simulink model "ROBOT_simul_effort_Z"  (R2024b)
settings: Solver=VariableStepAuto  StartTime=0.0  StopTime=5  RelTol=1e-3
undefined symbols (not defined in the file): a, ARRIERE_Defaut_sldprt, avant01_Defaut_sldprt, avant02_Defaut_sldprt, avant03_Defaut_sldprt, avant1_Defaut_sldprt, AXE, BASE_Defaut_sldprt, BIELLE, BIELLE_Defaut_sldprt, BRAS_Defaut_sldprt, bras_Defaut_sldprt, C_Realiste_sldprt, CABLE_Defaut_sldprt, cable_Defaut_sldprt, CACHE_Defaut_sldprt, CARTE, carte_Defaut_sldprt, CARTER, carter, CHC, CODEUR_Defaut_sldprt, cruciforme, cylindrique, deg, Drive, Fichiers, Fichiers_Matlab_sujetA, FIXATION, fixation_Defaut_sldprt, H, HEXAGONALE_Defaut_sldprt, joint_Defaut_sldprt, kg, m, M4, M4_Defaut_sldprt, manette1_Defaut_sldprt, manette2_Defaut_sldprt, MATLAB, Matlab, matlab_Defaut_sldprt, mm, modif, MOTEUR_Defaut_sldprt, N, NEZ_Defaut_sldprt, nom, palier, PARALLELOGRAMME_Defaut_sldprt, petite, plaque, rad, Ressort, Rondelle, ROTOR_Defaut_sldprt, s, SET, simple, socle_Defaut_sldprt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
libraries: sm_lib x463, fl_lib x45, nesl_utility x27, simulink x2
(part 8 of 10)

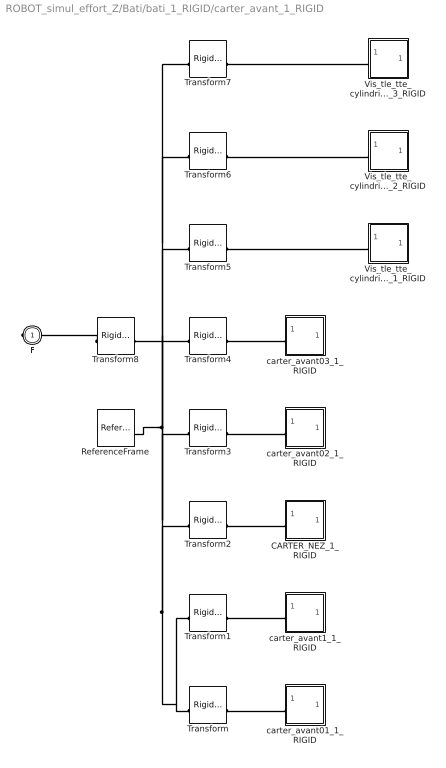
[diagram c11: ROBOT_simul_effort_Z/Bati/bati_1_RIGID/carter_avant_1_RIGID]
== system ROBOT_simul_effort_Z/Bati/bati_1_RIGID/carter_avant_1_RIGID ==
  CARTER_NEZ_1_RIGID : Subsystem
  ReferenceFrame : sm_lib/Frames and Transforms/Reference Frame
  Transform : sm_lib/Frames and Transforms/Rigid Transform  RotationMethod=None  FollAlignAxisA=+X  BaseAlignAxisA=+Y  FollAlignAxisB=+Y  BaseAlignAxisB=+Z  RotationStandardAxis=+Z  RotationAngle=0  RotationAngleUnits=deg  RotationArbitraryAxis=[0 0 1]  RotationSequenceAxes=FollowerAxes  RotationSequence=XYX  RotationSequenceAngles=[0 0 0]  RotationSequenceAnglesUnits=deg  RotationMatrix=[1 0 0; 0 1 0; 0 0 1]  Quaternion=[1 0 0 0]  TranslationMethod=Cartesian  TranslationCartesianOffset=[-17.102622676542445 -113.90982355031112 -1.7985612998927536e-11]  TranslationCartesianOffsetUnits=mm  TranslationStandardAxis=+Z  TranslationStandardOffset=0  TranslationStandardOffsetUnits=mm  TranslationROffset=0  TranslationROffsetUnits=m  TranslationThetaOffset=0  TranslationThetaOffsetUnits=deg  TranslationZOffset=0  TranslationZOffsetUnits=m
  Transform1 : sm_lib/Frames and Transforms/Rigid Transform  RotationMethod=None  FollAlignAxisA=+X  BaseAlignAxisA=+Y  FollAlignAxisB=+Y  BaseAlignAxisB=+Z  RotationStandardAxis=+Z  RotationAngle=0  RotationAngleUnits=deg  RotationArbitraryAxis=[0 0 1]  RotationSequenceAxes=FollowerAxes  RotationSequence=XYX  RotationSequenceAngles=[0 0 0]  RotationSequenceAnglesUnits=deg  RotationMatrix=[1 0 0; 0 1 0; 0 0 1]  Quaternion=[1 0 0 0]  TranslationMethod=Cartesian  TranslationCartesianOffset=[-17.102622676541863 -113.90982355031173 -1.7985612998927536e-11]  TranslationCartesianOffsetUnits=mm  TranslationStandardAxis=+Z  TranslationStandardOffset=0  TranslationStandardOffsetUnits=mm  TranslationROffset=0  TranslationROffsetUnits=m  TranslationThetaOffset=0  TranslationThetaOffsetUnits=deg  TranslationZOffset=0  TranslationZOffsetUnits=m
  Transform2 : sm_lib/Frames and Transforms/Rigid Transform  RotationMethod=ArbitraryAxis  FollAlignAxisA=+X  BaseAlignAxisA=+Y  FollAlignAxisB=+Y  BaseAlignAxisB=+Z  RotationStandardAxis=+Z  RotationAngle=3.1415926535897931  RotationAngleUnits=rad  RotationArbitraryAxis=[0 0.70710678118654746 0.70710678118654757]  RotationSequenceAxes=FollowerAxes  RotationSequence=XYX  RotationSequenceAngles=[0 0 0]  RotationSequenceAnglesUnits=deg  RotationMatrix=[1 0 0; 0 1 0; 0 0 1]  Quaternion=[1 0 0 0]  TranslationMethod=None  TranslationCartesianOffset=[0 0 0]  TranslationCartesianOffsetUnits=m  TranslationStandardAxis=+Z  TranslationStandardOffset=0  TranslationStandardOffsetUnits=m  TranslationROffset=0  TranslationROffsetUnits=m  TranslationThetaOffset=0  TranslationThetaOffsetUnits=deg  TranslationZOffset=0  TranslationZOffsetUnits=m
  Transform3 : sm_lib/Frames and Transforms/Rigid Transform  RotationMethod=ArbitraryAxis  FollAlignAxisA=+X  BaseAlignAxisA=+Y  FollAlignAxisB=+Y  BaseAlignAxisB=+Z  RotationStandardAxis=+Z  RotationAngle=2.094395102393193  RotationAngleUnits=rad  RotationArbitraryAxis=[0 0 1]  RotationSequenceAxes=FollowerAxes  RotationSequence=XYX  RotationSequenceAngles=[0 0 0]  RotationSequenceAnglesUnits=deg  RotationMatrix=[1 0 0; 0 1 0; 0 0 1]  Quaternion=[1 0 0 0]  TranslationMethod=Cartesian  TranslationCartesianOffset=[82.706805109614251 58.965176449688634 -1.7985612998927536e-11]  TranslationCartesianOffsetUnits=mm  TranslationStandardAxis=+Z  TranslationStandardOffset=0  TranslationStandardOffsetUnits=mm  TranslationROffset=0  TranslationROffsetUnits=m  TranslationThetaOffset=0  TranslationThetaOffsetUnits=deg  TranslationZOffset=0  TranslationZOffsetUnits=m
  Transform4 : sm_lib/Frames and Transforms/Rigid Transform  RotationMethod=ArbitraryAxis  FollAlignAxisA=+X  BaseAlignAxisA=+Y  FollAlignAxisB=+Y  BaseAlignAxisB=+Z  RotationStandardAxis=+Z  RotationAngle=2.0943951023932006  RotationAngleUnits=rad  RotationArbitraryAxis=[-0 -0 -1]  RotationSequenceAxes=FollowerAxes  RotationSequence=XYX  RotationSequenceAngles=[0 0 0]  RotationSequenceAnglesUnits=deg  RotationMatrix=[1 0 0; 0 1 0; 0 0 1]  Quaternion=[1 0 0 0]  TranslationMethod=Cartesian  TranslationCartesianOffset=[-116.91205046269873 58.965176449689402 -1.7985612998927536e-11]  TranslationCartesianOffsetUnits=mm  TranslationStandardAxis=+Z  TranslationStandardOffset=0  TranslationStandardOffsetUnits=mm  TranslationROffset=0  TranslationROffsetUnits=m  TranslationThetaOffset=0  TranslationThetaOffsetUnits=deg  TranslationZOffset=0  TranslationZOffsetUnits=m
  Transform5 : sm_lib/Frames and Transforms/Rigid Transform  RotationMethod=ArbitraryAxis  FollAlignAxisA=+X  BaseAlignAxisA=+Y  FollAlignAxisB=+Y  BaseAlignAxisB=+Z  RotationStandardAxis=+Z  RotationAngle=1.5707963267948968  RotationAngleUnits=rad  RotationArbitraryAxis=[0 1 0]  RotationSequenceAxes=FollowerAxes  RotationSequence=XYX  RotationSequenceAngles=[0 0 0]  RotationSequenceAnglesUnits=deg  RotationMatrix=[1 0 0; 0 1 0; 0 0 1]  Quaternion=[1 0 0 0]  TranslationMethod=Cartesian  TranslationCartesianOffset=[-32.01022121330513 -41.991412127562512 96.999999999981995]  TranslationCartesianOffsetUnits=mm  TranslationStandardAxis=+Z  TranslationStandardOffset=0  TranslationStandardOffsetUnits=mm  TranslationROffset=0  TranslationROffsetUnits=m  TranslationThetaOffset=0  TranslationThetaOffsetUnits=deg  TranslationZOffset=0  TranslationZOffsetUnits=m
  Transform6 : sm_lib/Frames and Transforms/Rigid Transform  RotationMethod=ArbitraryAxis  FollAlignAxisA=+X  BaseAlignAxisA=+Y  FollAlignAxisB=+Y  BaseAlignAxisB=+Z  RotationStandardAxis=+Z  RotationAngle=1.5707963267948968  RotationAngleUnits=rad  RotationArbitraryAxis=[0 1 0]  RotationSequenceAxes=FollowerAxes  RotationSequence=XYX  RotationSequenceAngles=[0 0 0]  RotationSequenceAnglesUnits=deg  RotationMatrix=[1 0 0; 0 1 0; 0 0 1]  Quaternion=[1 0 0 0]  TranslationMethod=Cartesian  TranslationCartesianOffset=[-47.17507990239649 35.916329780570692 96.999999999981995]  TranslationCartesianOffsetUnits=mm  TranslationStandardAxis=+Z  TranslationStandardOffset=0  TranslationStandardOffsetUnits=mm  TranslationROffset=0  TranslationROffsetUnits=m  TranslationThetaOffset=0  TranslationThetaOffsetUnits=deg  TranslationZOffset=0  TranslationZOffsetUnits=m
  Transform7 : sm_lib/Frames and Transforms/Rigid Transform  RotationMethod=ArbitraryAxis  FollAlignAxisA=+X  BaseAlignAxisA=+Y  FollAlignAxisB=+Y  BaseAlignAxisB=+Z  RotationStandardAxis=+Z  RotationAngle=1.5707963267948968  RotationAngleUnits=rad  RotationArbitraryAxis=[0 1 0]  RotationSequenceAxes=FollowerAxes  RotationSequence=XYX  RotationSequenceAngles=[0 0 0]  RotationSequenceAnglesUnits=deg  RotationMatrix=[1 0 0; 0 1 0; 0 0 1]  Quaternion=[1 0 0 0]  TranslationMethod=Cartesian  TranslationCartesianOffset=[27.877433086074202 10.09561169605827 96.999999999981995]  TranslationCartesianOffsetUnits=mm  TranslationStandardAxis=+Z  TranslationStandardOffset=0  TranslationStandardOffsetUnits=mm  TranslationROffset=0  TranslationROffsetUnits=m  TranslationThetaOffset=0  TranslationThetaOffsetUnits=deg  TranslationZOffset=0  TranslationZOffsetUnits=m
  Transform8 : sm_lib/Frames and Transforms/Rigid Transform  RotationMethod=None  FollAlignAxisA=+X  BaseAlignAxisA=+Y  FollAlignAxisB=+Y  BaseAlignAxisB=+Z  RotationStandardAxis=+Z  RotationAngle=0  RotationAngleUnits=deg  RotationArbitraryAxis=[0 0 1]  RotationSequenceAxes=FollowerAxes  RotationSequence=XYX  RotationSequenceAngles=[0 0 0]  RotationSequenceAnglesUnits=deg  RotationMatrix=[1 0 0; 0 1 0; 0 0 1]  Quaternion=[1 0 0 0]  TranslationMethod=Cartesian  TranslationCartesianOffset=[17.102622676542548 113.90982355031109 24.00000000001798]  TranslationCartesianOffsetUnits=mm  TranslationStandardAxis=+Z  TranslationStandardOffset=0  TranslationStandardOffsetUnits=mm  TranslationROffset=0  TranslationROffsetUnits=m  TranslationThetaOffset=0  TranslationThetaOffsetUnits=deg  TranslationZOffset=0  TranslationZOffsetUnits=m
  Vis_tle_tte_cylindrique_cruciforme_H_29x13_C_1_RIGID : Subsystem
  Vis_tle_tte_cylindrique_cruciforme_H_29x13_C_2_RIGID : Subsystem
  Vis_tle_tte_cylindrique_cruciforme_H_29x13_C_3_RIGID : Subsystem
  carter_avant01_1_RIGID : Subsystem
  carter_avant02_1_RIGID : Subsystem
  carter_avant03_1_RIGID : Subsystem
  carter_avant1_1_RIGID : Subsystem
  F : PMIOPort  Side=Right
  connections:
  Transform/RConn1 -- carter_avant01_1_RIGID/LConn1
  Transform1/RConn1 -- carter_avant1_1_RIGID/LConn1
  CARTER_NEZ_1_RIGID/LConn1 -- Transform2/RConn1
  Transform3/RConn1 -- carter_avant02_1_RIGID/LConn1
  Transform4/RConn1 -- carter_avant03_1_RIGID/LConn1
  Transform5/RConn1 -- Vis_tle_tte_cylindrique_cruciforme_H_29x13_C_1_RIGID/LConn1
  Transform6/RConn1 -- Vis_tle_tte_cylindrique_cruciforme_H_29x13_C_2_RIGID/LConn1
  Transform7/RConn1 -- Vis_tle_tte_cylindrique_cruciforme_H_29x13_C_3_RIGID/LConn1
  Transform/LConn1 -- Transform6/LConn1 -- Transform7/LConn1 -- Transform5/LConn1 -- Transform4/LConn1 -- ReferenceFrame/RConn1 -- Transform8/RConn1 -- Transform3/LConn1 -- Transform2/LConn1 -- Transform1/LConn1
  Transform8/LConn1 -- F/RConn1

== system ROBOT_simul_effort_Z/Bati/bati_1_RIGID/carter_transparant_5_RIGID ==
  ReferenceFrame : sm_lib/Frames and Transforms/Reference Frame
  Transform : sm_lib/Frames and Transforms/Rigid Transform  RotationMethod=ArbitraryAxis  FollAlignAxisA=+X  BaseAlignAxisA=+Y  FollAlignAxisB=+Y  BaseAlignAxisB=+Z  RotationStandardAxis=+Z  RotationAngle=2.0943951023932001  RotationAngleUnits=rad  RotationArbitraryAxis=[-0 -0 -1]  RotationSequenceAxes=FollowerAxes  RotationSequence=XYX  RotationSequenceAngles=[0 0 0]  RotationSequenceAnglesUnits=deg  RotationMatrix=[1 0 0; 0 1 0; 0 0 1]  Quaternion=[1 0 0 0]  TranslationMethod=Cartesian  TranslationCartesianOffset=[-114.07592590479371 112.90132228455712 35.212494571905935]  TranslationCartesianOffsetUnits=mm  TranslationStandardAxis=+Z  TranslationStandardOffset=0  TranslationStandardOffsetUnits=mm  TranslationROffset=0  TranslationROffsetUnits=m  TranslationThetaOffset=0  TranslationThetaOffsetUnits=deg  TranslationZOffset=0  TranslationZOffsetUnits=m
  Transform1 : sm_lib/Frames and Transforms/Rigid Transform  RotationMethod=None  FollAlignAxisA=+X  BaseAlignAxisA=+Y  FollAlignAxisB=+Y  BaseAlignAxisB=+Z  RotationStandardAxis=+Z  RotationAngle=0  RotationAngleUnits=deg  RotationArbitraryAxis=[0 0 1]  RotationSequenceAxes=FollowerAxes  RotationSequence=XYX  RotationSequenceAngles=[0 0 0]  RotationSequenceAnglesUnits=deg  RotationMatrix=[1 0 0; 0 1 0; 0 0 1]  Quaternion=[1 0 0 0]  TranslationMethod=Cartesian  TranslationCartesianOffset=[-14.266498118637394 -59.973677715443351 35.212494571905921]  TranslationCartesianOffsetUnits=mm  TranslationStandardAxis=+Z  TranslationStandardOffset=0  TranslationStandardOffsetUnits=mm  TranslationROffset=0  TranslationROffsetUnits=m  TranslationThetaOffset=0  TranslationThetaOffsetUnits=deg  TranslationZOffset=0  TranslationZOffsetUnits=m
  Transform2 : sm_lib/Frames and Transforms/Rigid Transform  RotationMethod=ArbitraryAxis  FollAlignAxisA=+X  BaseAlignAxisA=+Y  FollAlignAxisB=+Y  BaseAlignAxisB=+Z  RotationStandardAxis=+Z  RotationAngle=2.0943951023931877  RotationAngleUnits=rad  RotationArbitraryAxis=[0 0 1]  RotationSequenceAxes=FollowerAxes  RotationSequence=XYX  RotationSequenceAngles=[0 0 0]  RotationSequenceAnglesUnits=deg  RotationMatrix=[1 0 0; 0 1 0; 0 0 1]  Quaternion=[1 0 0 0]  TranslationMethod=Cartesian  TranslationCartesianOffset=[85.542929667519687 112.90132228455593 35.212494571905921]  TranslationCartesianOffsetUnits=mm  TranslationStandardAxis=+Z  TranslationStandardOffset=0  TranslationStandardOffsetUnits=mm  TranslationROffset=0  TranslationROffsetUnits=m  TranslationThetaOffset=0  TranslationThetaOffsetUnits=deg  TranslationZOffset=0  TranslationZOffsetUnits=m
  Transform3 : sm_lib/Frames and Transforms/Rigid Transform  RotationMethod=ArbitraryAxis  FollAlignAxisA=+X  BaseAlignAxisA=+Y  FollAlignAxisB=+Y  BaseAlignAxisB=+Z  RotationStandardAxis=+Z  RotationAngle=0.025132741228718395  RotationAngleUnits=rad  RotationArbitraryAxis=[0 0 -1]  RotationSequenceAxes=FollowerAxes  RotationSequence=XYX  RotationSequenceAngles=[0 0 0]  RotationSequenceAnglesUnits=deg  RotationMatrix=[1 0 0; 0 1 0; 0 0 1]  Quaternion=[1 0 0 0]  TranslationMethod=Cartesian  TranslationCartesianOffset=[12.872893350874152 59.632616111037024 -35.212494571905921]  TranslationCartesianOffsetUnits=mm  TranslationStandardAxis=+Z  TranslationStandardOffset=0  TranslationStandardOffsetUnits=mm  TranslationROffset=0  TranslationROffsetUnits=m  TranslationThetaOffset=0  TranslationThetaOffsetUnits=deg  TranslationZOffset=0  TranslationZOffsetUnits=m
  carter_transparent2_1_RIGID : Subsystem
  carter_transparent_1_RIGID : Subsystem
  carter_transparent_modif_matlab_1_RIGID : Subsystem
  F : PMIOPort  Side=Right
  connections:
  Transform/RConn1 -- carter_transparent_1_RIGID/LConn1
  Transform1/RConn1 -- carter_transparent2_1_RIGID/LConn1
  Transform2/RConn1 -- carter_transparent_modif_matlab_1_RIGID/LConn1
  Transform/LConn1 -- Transform1/LConn1 -- Transform2/LConn1 -- ReferenceFrame/RConn1 -- Transform3/RConn1
  Transform3/LConn1 -- F/RConn1

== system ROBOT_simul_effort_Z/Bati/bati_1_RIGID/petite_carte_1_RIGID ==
  ReferenceFrame : sm_lib/Frames and Transforms/Reference Frame
  Solid : sm_lib/Body Elements/File Solid  ExtGeomFileName=/MATLAB Drive/Fichiers_Matlab_sujetA/Fichiers Matlab/STL/petite carte_Defaut_sldprt.STL  UnitType=Custom  ExtGeomFileUnits=mm  StepReaderType=HEX  ExportConvexHullGeometry=off  InertiaType=Custom  BasedOnType=Density  Density=1000  DensityUnits=kg/(m^3)  Mass=0.00048082183649251445  MassUnits=kg  CenterOfMass=[19.91458998704724 1.4286045215267169 0.6668228749994265]  CenterOfMassUnits=mm  MomentsOfInertia=[0.0075326471062909569 0.048633515547401453 0.053492974016950315]  MomentsOfInertiaUnits=kg*mm^2  ProductsOfInertia=[9.9546833043094831e-05 0.0011485008863759011 0.0086575785704640102]  ProductsOfInertiaUnits=kg*mm^2  GraphicType=FromGeometry  MarkerShape=Sphere  MarkerSize=10  GraphicVisPropType=SimpleVisualProperties  GraphicDiffuseColor=[0 0.50196078431372548 0]  GraphicOpacity=1  GraphicSpecularColor=[0.5 0.5 0.5 1.0]  GraphicAmbientColor=[0.15 0.15 0.15 1.0]  GraphicEmissiveColor=[0.0 0.0 0.0 1.0]  GraphicShininess=75  DoExposeReferenceFrame=on  SerializedFrames=<Frames/>
  F : PMIOPort  Side=Left
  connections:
  Solid/RConn1 -- ReferenceFrame/RConn1 -- F/RConn1

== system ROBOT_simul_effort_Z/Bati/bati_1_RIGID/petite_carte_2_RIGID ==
  ReferenceFrame : sm_lib/Frames and Transforms/Reference Frame
  Solid : sm_lib/Body Elements/File Solid  ExtGeomFileName=/MATLAB Drive/Fichiers_Matlab_sujetA/Fichiers Matlab/STL/petite carte_Defaut_sldprt.STL  UnitType=Custom  ExtGeomFileUnits=mm  StepReaderType=HEX  ExportConvexHullGeometry=off  InertiaType=Custom  BasedOnType=Density  Density=1000  DensityUnits=kg/(m^3)  Mass=0.00048082183649251445  MassUnits=kg  CenterOfMass=[19.91458998704724 1.4286045215267169 0.6668228749994265]  CenterOfMassUnits=mm  MomentsOfInertia=[0.0075326471062909569 0.048633515547401453 0.053492974016950315]  MomentsOfInertiaUnits=kg*mm^2  ProductsOfInertia=[9.9546833043094831e-05 0.0011485008863759011 0.0086575785704640102]  ProductsOfInertiaUnits=kg*mm^2  GraphicType=FromGeometry  MarkerShape=Sphere  MarkerSize=10  GraphicVisPropType=SimpleVisualProperties  GraphicDiffuseColor=[0 0.50196078431372548 0]  GraphicOpacity=1  GraphicSpecularColor=[0.5 0.5 0.5 1.0]  GraphicAmbientColor=[0.15 0.15 0.15 1.0]  GraphicEmissiveColor=[0.0 0.0 0.0 1.0]  GraphicShininess=75  DoExposeReferenceFrame=on  SerializedFrames=<Frames/>
  F : PMIOPort  Side=Left
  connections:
  Solid/RConn1 -- ReferenceFrame/RConn1 -- F/RConn1

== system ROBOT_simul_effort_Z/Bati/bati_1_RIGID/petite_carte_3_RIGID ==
  ReferenceFrame : sm_lib/Frames and Transforms/Reference Frame
  Solid : sm_lib/Body Elements/File Solid  ExtGeomFileName=/MATLAB Drive/Fichiers_Matlab_sujetA/Fichiers Matlab/STL/petite carte_Defaut_sldprt.STL  UnitType=Custom  ExtGeomFileUnits=mm  StepReaderType=HEX  ExportConvexHullGeometry=off  InertiaType=Custom  BasedOnType=Density  Density=1000  DensityUnits=kg/(m^3)  Mass=0.00048082183649251445  MassUnits=kg  CenterOfMass=[19.91458998704724 1.4286045215267169 0.6668228749994265]  CenterOfMassUnits=mm  MomentsOfInertia=[0.0075326471062909569 0.048633515547401453 0.053492974016950315]  MomentsOfInertiaUnits=kg*mm^2  ProductsOfInertia=[9.9546833043094831e-05 0.0011485008863759011 0.0086575785704640102]  ProductsOfInertiaUnits=kg*mm^2  GraphicType=FromGeometry  MarkerShape=Sphere  MarkerSize=10  GraphicVisPropType=SimpleVisualProperties  GraphicDiffuseColor=[0 0.50196078431372548 0]  GraphicOpacity=1  GraphicSpecularColor=[0.5 0.5 0.5 1.0]  GraphicAmbientColor=[0.15 0.15 0.15 1.0]  GraphicEmissiveColor=[0.0 0.0 0.0 1.0]  GraphicShininess=75  DoExposeReferenceFrame=on  SerializedFrames=<Frames/>
  F : PMIOPort  Side=Left
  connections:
  Solid/RConn1 -- ReferenceFrame/RConn1 -- F/RConn1

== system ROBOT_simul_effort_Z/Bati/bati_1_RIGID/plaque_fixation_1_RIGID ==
  ReferenceFrame : sm_lib/Frames and Transforms/Reference Frame
  Solid : sm_lib/Body Elements/File Solid  ExtGeomFileName=/MATLAB Drive/Fichiers_Matlab_sujetA/Fichiers Matlab/STL/plaque fixation_Defaut_sldprt.STL  UnitType=Custom  ExtGeomFileUnits=mm  StepReaderType=HEX  ExportConvexHullGeometry=off  InertiaType=Custom  BasedOnType=Density  Density=1000  DensityUnits=kg/(m^3)  Mass=0.13619587212093154  MassUnits=kg  CenterOfMass=[0 57.644814512190067 6.7752904956014124]  CenterOfMassUnits=mm  MomentsOfInertia=[230.56748251711528 59.503021506275417 273.91192419339654]  MomentsOfInertiaUnits=kg*mm^2  ProductsOfInertia=[16.91481201365259 0 0]  ProductsOfInertiaUnits=kg*mm^2  GraphicType=FromGeometry  MarkerShape=Sphere  MarkerSize=10  GraphicVisPropType=SimpleVisualProperties  GraphicDiffuseColor=[0.6470588235294118 0.61960784313725492 0.58823529411764708]  GraphicOpacity=1  GraphicSpecularColor=[0.5 0.5 0.5 1.0]  GraphicAmbientColor=[0.15 0.15 0.15 1.0]  GraphicEmissiveColor=[0.0 0.0 0.0 1.0]  GraphicShininess=75  DoExposeReferenceFrame=on  SerializedFrames=<Frames/>
  F : PMIOPort  Side=Left
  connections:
  Solid/RConn1 -- ReferenceFrame/RConn1 -- F/RConn1

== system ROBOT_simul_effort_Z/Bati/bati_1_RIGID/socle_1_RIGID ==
  ReferenceFrame : sm_lib/Frames and Transforms/Reference Frame
  Solid : sm_lib/Body Elements/File Solid  ExtGeomFileName=/MATLAB Drive/Fichiers_Matlab_sujetA/Fichiers Matlab/STL/socle_Defaut_sldprt.STL  UnitType=Custom  ExtGeomFileUnits=mm  StepReaderType=HEX  ExportConvexHullGeometry=off  InertiaType=Custom  BasedOnType=Density  Density=1000  DensityUnits=kg/(m^3)  Mass=0.22494978957848721  MassUnits=kg  CenterOfMass=[-0.04792533570938888 16.018647482078187 6.7264124950212594]  CenterOfMassUnits=mm  MomentsOfInertia=[992.11143480501664 1618.7630611955949 2601.3810500563377]  MomentsOfInertiaUnits=kg*mm^2  ProductsOfInertia=[-5.1990662975402211 -0.041150083489637494 0.38689094335060764]  ProductsOfInertiaUnits=kg*mm^2  GraphicType=FromGeometry  MarkerShape=Sphere  MarkerSize=10  GraphicVisPropType=SimpleVisualProperties  GraphicDiffuseColor=[0.792156862745098 0.81960784313725488 0.93333333333333335]  GraphicOpacity=1  GraphicSpecularColor=[0.5 0.5 0.5 1.0]  GraphicAmbientColor=[0.15 0.15 0.15 1.0]  GraphicEmissiveColor=[0.0 0.0 0.0 1.0]  GraphicShininess=75  DoExposeReferenceFrame=on  SerializedFrames=<Frames/>
  F : PMIOPort  Side=Left
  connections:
  Solid/RConn1 -- ReferenceFrame/RConn1 -- F/RConn1

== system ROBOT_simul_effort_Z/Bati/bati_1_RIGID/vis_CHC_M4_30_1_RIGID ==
  ReferenceFrame : sm_lib/Frames and Transforms/Reference Frame
  Solid : sm_lib/Body Elements/File Solid  ExtGeomFileName=/MATLAB Drive/Fichiers_Matlab_sujetA/Fichiers Matlab/STL/vis CHC M4-30_Defaut_sldprt.STL  UnitType=Custom  ExtGeomFileUnits=mm  StepReaderType=HEX  ExportConvexHullGeometry=off  InertiaType=Custom  BasedOnType=Density  Density=1000  DensityUnits=kg/(m^3)  Mass=0.00050829612748328964  MassUnits=kg  CenterOfMass=[0 0 19.413574172112984]  CenterOfMassUnits=mm  MomentsOfInertia=[0.056747582392929367 0.056747582392929367 0.0016443905083794684]  MomentsOfInertiaUnits=kg*mm^2  ProductsOfInertia=[0 0 0]  ProductsOfInertiaUnits=kg*mm^2  GraphicType=FromGeometry  MarkerShape=Sphere  MarkerSize=10  GraphicVisPropType=SimpleVisualProperties  GraphicDiffuseColor=[0.75294117647058822 0.75294117647058822 0.75294117647058822]  GraphicOpacity=1  GraphicSpecularColor=[0.5 0.5 0.5 1.0]  GraphicAmbientColor=[0.15 0.15 0.15 1.0]  GraphicEmissiveColor=[0.0 0.0 0.0 1.0]  GraphicShininess=75  DoExposeReferenceFrame=on  SerializedFrames=<Frames/>
  F : PMIOPort  Side=Left
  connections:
  Solid/RConn1 -- ReferenceFrame/RConn1 -- F/RConn1

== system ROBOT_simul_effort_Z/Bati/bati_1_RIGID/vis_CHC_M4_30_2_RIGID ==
  ReferenceFrame : sm_lib/Frames and Transforms/Reference Frame
  Solid : sm_lib/Body Elements/File Solid  ExtGeomFileName=/MATLAB Drive/Fichiers_Matlab_sujetA/Fichiers Matlab/STL/vis CHC M4-30_Defaut_sldprt.STL  UnitType=Custom  ExtGeomFileUnits=mm  StepReaderType=HEX  ExportConvexHullGeometry=off  InertiaType=Custom  BasedOnType=Density  Density=1000  DensityUnits=kg/(m^3)  Mass=0.00050829612748328964  MassUnits=kg  CenterOfMass=[0 0 19.413574172112984]  CenterOfMassUnits=mm  MomentsOfInertia=[0.056747582392929367 0.056747582392929367 0.0016443905083794684]  MomentsOfInertiaUnits=kg*mm^2  ProductsOfInertia=[0 0 0]  ProductsOfInertiaUnits=kg*mm^2  GraphicType=FromGeometry  MarkerShape=Sphere  MarkerSize=10  GraphicVisPropType=SimpleVisualProperties  GraphicDiffuseColor=[0.75294117647058822 0.75294117647058822 0.75294117647058822]  GraphicOpacity=1  GraphicSpecularColor=[0.5 0.5 0.5 1.0]  GraphicAmbientColor=[0.15 0.15 0.15 1.0]  GraphicEmissiveColor=[0.0 0.0 0.0 1.0]  GraphicShininess=75  DoExposeReferenceFrame=on  SerializedFrames=<Frames/>
  F : PMIOPort  Side=Left
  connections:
  Solid/RConn1 -- ReferenceFrame/RConn1 -- F/RConn1

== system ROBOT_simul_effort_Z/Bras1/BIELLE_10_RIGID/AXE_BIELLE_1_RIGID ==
  ReferenceFrame : sm_lib/Frames and Transforms/Reference Frame
  Solid : sm_lib/Body Elements/File Solid  ExtGeomFileName=/MATLAB Drive/Fichiers_Matlab_sujetA/Fichiers Matlab/STL/AXE BIELLE_Defaut_sldprt.STL  UnitType=Custom  ExtGeomFileUnits=mm  StepReaderType=HEX  ExportConvexHullGeometry=off  InertiaType=Custom  BasedOnType=Density  Density=1000  DensityUnits=kg/(m^3)  Mass=0.0008880235381781051  MassUnits=kg  CenterOfMass=[0 0 0]  CenterOfMassUnits=mm  MomentsOfInertia=[0.018768660222737772 0.018768660222737772 0.0009874025874388381]  MomentsOfInertiaUnits=kg*mm^2  ProductsOfInertia=[0 0 0]  ProductsOfInertiaUnits=kg*mm^2  GraphicType=FromGeometry  MarkerShape=Sphere  MarkerSize=10  GraphicVisPropType=SimpleVisualProperties  GraphicDiffuseColor=[1 0.94901960784313721 0.90980392156862744]  GraphicOpacity=1  GraphicSpecularColor=[0.5 0.5 0.5 1.0]  GraphicAmbientColor=[0.15 0.15 0.15 1.0]  GraphicEmissiveColor=[0.0 0.0 0.0 1.0]  GraphicShininess=75  DoExposeReferenceFrame=on  SerializedFrames=<Frames/>
  F : PMIOPort  Side=Left
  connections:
  Solid/RConn1 -- ReferenceFrame/RConn1 -- F/RConn1

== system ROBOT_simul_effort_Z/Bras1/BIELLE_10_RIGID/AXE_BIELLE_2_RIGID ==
  ReferenceFrame : sm_lib/Frames and Transforms/Reference Frame
  Solid : sm_lib/Body Elements/File Solid  ExtGeomFileName=/MATLAB Drive/Fichiers_Matlab_sujetA/Fichiers Matlab/STL/AXE BIELLE_Defaut_sldprt.STL  UnitType=Custom  ExtGeomFileUnits=mm  StepReaderType=HEX  ExportConvexHullGeometry=off  InertiaType=Custom  BasedOnType=Density  Density=1000  DensityUnits=kg/(m^3)  Mass=0.0008880235381781051  MassUnits=kg  CenterOfMass=[0 0 0]  CenterOfMassUnits=mm  MomentsOfInertia=[0.018768660222737772 0.018768660222737772 0.0009874025874388381]  MomentsOfInertiaUnits=kg*mm^2  ProductsOfInertia=[0 0 0]  ProductsOfInertiaUnits=kg*mm^2  GraphicType=FromGeometry  MarkerShape=Sphere  MarkerSize=10  GraphicVisPropType=SimpleVisualProperties  GraphicDiffuseColor=[1 0.94901960784313721 0.90980392156862744]  GraphicOpacity=1  GraphicSpecularColor=[0.5 0.5 0.5 1.0]  GraphicAmbientColor=[0.15 0.15 0.15 1.0]  GraphicEmissiveColor=[0.0 0.0 0.0 1.0]  GraphicShininess=75  DoExposeReferenceFrame=on  SerializedFrames=<Frames/>
  F : PMIOPort  Side=Left
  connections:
  Solid/RConn1 -- ReferenceFrame/RConn1 -- F/RConn1

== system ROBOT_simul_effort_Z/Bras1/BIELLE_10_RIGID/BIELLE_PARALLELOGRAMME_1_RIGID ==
  ReferenceFrame : sm_lib/Frames and Transforms/Reference Frame
  Solid : sm_lib/Body Elements/File Solid  ExtGeomFileName=/MATLAB Drive/Fichiers_Matlab_sujetA/Fichiers Matlab/STL/BIELLE PARALLELOGRAMME_Defaut_sldprt.STL  UnitType=Custom  ExtGeomFileUnits=mm  StepReaderType=HEX  ExportConvexHullGeometry=off  InertiaType=Custom  BasedOnType=Density  Density=1000  DensityUnits=kg/(m^3)  Mass=0.0079529027635324764  MassUnits=kg  CenterOfMass=[0 3.1653377955585489 0]  CenterOfMassUnits=mm  MomentsOfInertia=[7.7987017961340088 7.8475939194203406 0.14816857834406802]  MomentsOfInertiaUnits=kg*mm^2  ProductsOfInertia=[0 0 0]  ProductsOfInertiaUnits=kg*mm^2  GraphicType=FromGeometry  MarkerShape=Sphere  MarkerSize=10  GraphicVisPropType=SimpleVisualProperties  GraphicDiffuseColor=[0.6 1.0 1.0]  GraphicOpacity=1  GraphicSpecularColor=[0.5 0.5 0.5 1.0]  GraphicAmbientColor=[0.15 0.15 0.15 1.0]  GraphicEmissiveColor=[0.0 0.0 0.0 1.0]  GraphicShininess=75  DoExposeReferenceFrame=on  SerializedFrames=<Frames/>
  F : PMIOPort  Side=Left
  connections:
  Solid/RConn1 -- ReferenceFrame/RConn1 -- F/RConn1

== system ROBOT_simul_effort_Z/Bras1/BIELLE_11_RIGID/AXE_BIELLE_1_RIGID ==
  ReferenceFrame : sm_lib/Frames and Transforms/Reference Frame
  Solid : sm_lib/Body Elements/File Solid  ExtGeomFileName=/MATLAB Drive/Fichiers_Matlab_sujetA/Fichiers Matlab/STL/AXE BIELLE_Defaut_sldprt.STL  UnitType=Custom  ExtGeomFileUnits=mm  StepReaderType=HEX  ExportConvexHullGeometry=off  InertiaType=Custom  BasedOnType=Density  Density=1000  DensityUnits=kg/(m^3)  Mass=0.0008880235381781051  MassUnits=kg  CenterOfMass=[0 0 0]  CenterOfMassUnits=mm  MomentsOfInertia=[0.018768660222737772 0.018768660222737772 0.0009874025874388381]  MomentsOfInertiaUnits=kg*mm^2  ProductsOfInertia=[0 0 0]  ProductsOfInertiaUnits=kg*mm^2  GraphicType=FromGeometry  MarkerShape=Sphere  MarkerSize=10  GraphicVisPropType=SimpleVisualProperties  GraphicDiffuseColor=[1 0.94901960784313721 0.90980392156862744]  GraphicOpacity=1  GraphicSpecularColor=[0.5 0.5 0.5 1.0]  GraphicAmbientColor=[0.15 0.15 0.15 1.0]  GraphicEmissiveColor=[0.0 0.0 0.0 1.0]  GraphicShininess=75  DoExposeReferenceFrame=on  SerializedFrames=<Frames/>
  F : PMIOPort  Side=Left
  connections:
  Solid/RConn1 -- ReferenceFrame/RConn1 -- F/RConn1

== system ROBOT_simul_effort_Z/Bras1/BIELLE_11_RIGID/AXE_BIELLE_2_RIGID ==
  ReferenceFrame : sm_lib/Frames and Transforms/Reference Frame
  Solid : sm_lib/Body Elements/File Solid  ExtGeomFileName=/MATLAB Drive/Fichiers_Matlab_sujetA/Fichiers Matlab/STL/AXE BIELLE_Defaut_sldprt.STL  UnitType=Custom  ExtGeomFileUnits=mm  StepReaderType=HEX  ExportConvexHullGeometry=off  InertiaType=Custom  BasedOnType=Density  Density=1000  DensityUnits=kg/(m^3)  Mass=0.0008880235381781051  MassUnits=kg  CenterOfMass=[0 0 0]  CenterOfMassUnits=mm  MomentsOfInertia=[0.018768660222737772 0.018768660222737772 0.0009874025874388381]  MomentsOfInertiaUnits=kg*mm^2  ProductsOfInertia=[0 0 0]  ProductsOfInertiaUnits=kg*mm^2  GraphicType=FromGeometry  MarkerShape=Sphere  MarkerSize=10  GraphicVisPropType=SimpleVisualProperties  GraphicDiffuseColor=[1 0.94901960784313721 0.90980392156862744]  GraphicOpacity=1  GraphicSpecularColor=[0.5 0.5 0.5 1.0]  GraphicAmbientColor=[0.15 0.15 0.15 1.0]  GraphicEmissiveColor=[0.0 0.0 0.0 1.0]  GraphicShininess=75  DoExposeReferenceFrame=on  SerializedFrames=<Frames/>
  F : PMIOPort  Side=Left
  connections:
  Solid/RConn1 -- ReferenceFrame/RConn1 -- F/RConn1

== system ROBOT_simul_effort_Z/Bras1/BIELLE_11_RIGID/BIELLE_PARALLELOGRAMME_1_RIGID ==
  ReferenceFrame : sm_lib/Frames and Transforms/Reference Frame
  Solid : sm_lib/Body Elements/File Solid  ExtGeomFileName=/MATLAB Drive/Fichiers_Matlab_sujetA/Fichiers Matlab/STL/BIELLE PARALLELOGRAMME_Defaut_sldprt.STL  UnitType=Custom  ExtGeomFileUnits=mm  StepReaderType=HEX  ExportConvexHullGeometry=off  InertiaType=Custom  BasedOnType=Density  Density=1000  DensityUnits=kg/(m^3)  Mass=0.0079529027635324764  MassUnits=kg  CenterOfMass=[0 3.1653377955585489 0]  CenterOfMassUnits=mm  MomentsOfInertia=[7.7987017961340088 7.8475939194203406 0.14816857834406802]  MomentsOfInertiaUnits=kg*mm^2  ProductsOfInertia=[0 0 0]  ProductsOfInertiaUnits=kg*mm^2  GraphicType=FromGeometry  MarkerShape=Sphere  MarkerSize=10  GraphicVisPropType=SimpleVisualProperties  GraphicDiffuseColor=[0.6 1.0 1.0]  GraphicOpacity=1  GraphicSpecularColor=[0.5 0.5 0.5 1.0]  GraphicAmbientColor=[0.15 0.15 0.15 1.0]  GraphicEmissiveColor=[0.0 0.0 0.0 1.0]  GraphicShininess=75  DoExposeReferenceFrame=on  SerializedFrames=<Frames/>
  F : PMIOPort  Side=Left
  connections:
  Solid/RConn1 -- ReferenceFrame/RConn1 -- F/RConn1

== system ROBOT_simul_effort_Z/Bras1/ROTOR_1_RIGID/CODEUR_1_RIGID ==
  ReferenceFrame : sm_lib/Frames and Transforms/Reference Frame
  Solid : sm_lib/Body Elements/File Solid  ExtGeomFileName=/MATLAB Drive/Fichiers_Matlab_sujetA/Fichiers Matlab/STL/CODEUR_Defaut_sldprt.STL  UnitType=Custom  ExtGeomFileUnits=mm  StepReaderType=HEX  ExportConvexHullGeometry=off  InertiaType=Custom  BasedOnType=Density  Density=1000  DensityUnits=kg/(m^3)  Mass=0.0064318274490095598  MassUnits=kg  CenterOfMass=[0 6.0527709306807029 -0.1964144966449296]  CenterOfMassUnits=mm  MomentsOfInertia=[0.92812714377460337 1.2443807481520079 0.93469179577802664]  MomentsOfInertiaUnits=kg*mm^2  ProductsOfInertia=[0.0063987198741970201 0 0]  ProductsOfInertiaUnits=kg*mm^2  GraphicType=FromGeometry  MarkerShape=Sphere  MarkerSize=10  GraphicVisPropType=SimpleVisualProperties  GraphicDiffuseColor=[0.2 1.0 0.0]  GraphicOpacity=1  GraphicSpecularColor=[0.5 0.5 0.5 1.0]  GraphicAmbientColor=[0.15 0.15 0.15 1.0]  GraphicEmissiveColor=[0.0 0.0 0.0 1.0]  GraphicShininess=75  DoExposeReferenceFrame=on  SerializedFrames=<Frames/>
  F : PMIOPort  Side=Left
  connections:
  Solid/RConn1 -- ReferenceFrame/RConn1 -- F/RConn1

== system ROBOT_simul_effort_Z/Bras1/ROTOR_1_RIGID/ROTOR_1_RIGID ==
  ReferenceFrame : sm_lib/Frames and Transforms/Reference Frame
  Solid : sm_lib/Body Elements/File Solid  ExtGeomFileName=/MATLAB Drive/Fichiers_Matlab_sujetA/Fichiers Matlab/STL/ROTOR_Defaut_sldprt.STL  UnitType=Custom  ExtGeomFileUnits=mm  StepReaderType=HEX  ExportConvexHullGeometry=off  InertiaType=Custom  BasedOnType=Density  Density=1000  DensityUnits=kg/(m^3)  Mass=0.07643998420030651  MassUnits=kg  CenterOfMass=[0 30.928341108151987 -0.0018262913863015125]  CenterOfMassUnits=mm  MomentsOfInertia=[14.640748377051393 9.6696912582654697 14.640902193857929]  MomentsOfInertiaUnits=kg*mm^2  ProductsOfInertia=[0.0065014820412302417 0 0]  ProductsOfInertiaUnits=kg*mm^2  GraphicType=FromGeometry  MarkerShape=Sphere  MarkerSize=10  GraphicVisPropType=SimpleVisualProperties  GraphicDiffuseColor=[0.53725490196078429 0.34901960784313724 0.33725490196078434]  GraphicOpacity=1  GraphicSpecularColor=[0.5 0.5 0.5 1.0]  GraphicAmbientColor=[0.15 0.15 0.15 1.0]  GraphicEmissiveColor=[0.0 0.0 0.0 1.0]  GraphicShininess=75  DoExposeReferenceFrame=on  SerializedFrames=<Frames/>
  F : PMIOPort  Side=Left
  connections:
  Solid/RConn1 -- ReferenceFrame/RConn1 -- F/RConn1

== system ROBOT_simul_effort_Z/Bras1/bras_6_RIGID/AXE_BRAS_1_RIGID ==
  ReferenceFrame : sm_lib/Frames and Transforms/Reference Frame
  Solid : sm_lib/Body Elements/File Solid  ExtGeomFileName=/MATLAB Drive/Fichiers_Matlab_sujetA/Fichiers Matlab/STL/AXE BRAS_Defaut_sldprt.STL  UnitType=Custom  ExtGeomFileUnits=mm  StepReaderType=HEX  ExportConvexHullGeometry=off  InertiaType=Custom  BasedOnType=Density  Density=1000  DensityUnits=kg/(m^3)  Mass=0.0015327306958088996  MassUnits=kg  CenterOfMass=[0 0 0]  CenterOfMassUnits=mm  MomentsOfInertia=[0.11359646260705632 0.11359646260705632 0.0017137152305883286]  MomentsOfInertiaUnits=kg*mm^2  ProductsOfInertia=[0 0 0]  ProductsOfInertiaUnits=kg*mm^2  GraphicType=FromGeometry  MarkerShape=Sphere  MarkerSize=10  GraphicVisPropType=SimpleVisualProperties  GraphicDiffuseColor=[0.6470588235294118 0.61960784313725492 0.58823529411764708]  GraphicOpacity=1  GraphicSpecularColor=[0.5 0.5 0.5 1.0]  GraphicAmbientColor=[0.15 0.15 0.15 1.0]  GraphicEmissiveColor=[0.0 0.0 0.0 1.0]  GraphicShininess=75  DoExposeReferenceFrame=on  SerializedFrames=<Frames/>
  F : PMIOPort  Side=Left
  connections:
  Solid/RConn1 -- ReferenceFrame/RConn1 -- F/RConn1

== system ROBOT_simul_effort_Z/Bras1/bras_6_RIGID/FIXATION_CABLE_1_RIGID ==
  ReferenceFrame : sm_lib/Frames and Transforms/Reference Frame
  Solid : sm_lib/Body Elements/File Solid  ExtGeomFileName=/MATLAB Drive/Fichiers_Matlab_sujetA/Fichiers Matlab/STL/FIXATION CABLE_Defaut_sldprt.STL  UnitType=Custom  ExtGeomFileUnits=mm  StepReaderType=HEX  ExportConvexHullGeometry=off  InertiaType=Custom  BasedOnType=Density  Density=1000  DensityUnits=kg/(m^3)  Mass=3.2000000000000007e-06  MassUnits=kg  CenterOfMass=[0 0 0.099999999999999992]  CenterOfMassUnits=mm  MomentsOfInertia=[4.2773333333333348e-06 4.2773333333333331e-06 8.5333333333333352e-06]  MomentsOfInertiaUnits=kg*mm^2  ProductsOfInertia=[0 0 0]  ProductsOfInertiaUnits=kg*mm^2  GraphicType=FromGeometry  MarkerShape=Sphere  MarkerSize=10  GraphicVisPropType=SimpleVisualProperties  GraphicDiffuseColor=[0.25098039215686274 0.25098039215686274 0.25098039215686274]  GraphicOpacity=1  GraphicSpecularColor=[0.5 0.5 0.5 1.0]  GraphicAmbientColor=[0.15 0.15 0.15 1.0]  GraphicEmissiveColor=[0.0 0.0 0.0 1.0]  GraphicShininess=75  DoExposeReferenceFrame=on  SerializedFrames=<Frames/>
  F : PMIOPort  Side=Left
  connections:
  Solid/RConn1 -- ReferenceFrame/RConn1 -- F/RConn1

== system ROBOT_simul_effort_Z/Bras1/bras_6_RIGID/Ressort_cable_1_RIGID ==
  ReferenceFrame : sm_lib/Frames and Transforms/Reference Frame
  Solid : sm_lib/Body Elements/File Solid  ExtGeomFileName=/MATLAB Drive/Fichiers_Matlab_sujetA/Fichiers Matlab/STL/Ressort cable_Defaut_sldprt.STL  UnitType=Custom  ExtGeomFileUnits=mm  StepReaderType=HEX  ExportConvexHullGeometry=off  InertiaType=Custom  BasedOnType=Density  Density=1000  DensityUnits=kg/(m^3)  Mass=0.0011765814520035881  MassUnits=kg  CenterOfMass=[0.086849073647483815 -0.00090479521327996976 6.9508776157243597]  CenterOfMassUnits=mm  MomentsOfInertia=[0.034952381374405594 0.034338972761516762 0.0097063586011258158]  MomentsOfInertiaUnits=kg*mm^2  ProductsOfInertia=[0.00037229322226744533 1.6947615167207185e-06 2.0937803976811866e-06]  ProductsOfInertiaUnits=kg*mm^2  GraphicType=FromGeometry  MarkerShape=Sphere  MarkerSize=10  GraphicVisPropType=SimpleVisualProperties  GraphicDiffuseColor=[0.0 0.0 0.0]  GraphicOpacity=1  GraphicSpecularColor=[0.5 0.5 0.5 1.0]  GraphicAmbientColor=[0.15 0.15 0.15 1.0]  GraphicEmissiveColor=[0.0 0.0 0.0 1.0]  GraphicShininess=75  DoExposeReferenceFrame=on  SerializedFrames=<Frames/>
  F : PMIOPort  Side=Left
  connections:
  Solid/RConn1 -- ReferenceFrame/RConn1 -- F/RConn1

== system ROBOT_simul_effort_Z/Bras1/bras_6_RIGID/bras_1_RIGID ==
  ReferenceFrame : sm_lib/Frames and Transforms/Reference Frame
  Solid : sm_lib/Body Elements/File Solid  ExtGeomFileName=/MATLAB Drive/Fichiers_Matlab_sujetA/Fichiers Matlab/STL/bras_Defaut_sldprt.STL  UnitType=Custom  ExtGeomFileUnits=mm  StepReaderType=HEX  ExportConvexHullGeometry=off  InertiaType=Custom  BasedOnType=Density  Density=1000  DensityUnits=kg/(m^3)  Mass=0.06566875822643542  MassUnits=kg  CenterOfMass=[23.925748169887701 -4.7774352723885904 0.0071346362933715022]  CenterOfMassUnits=mm  MomentsOfInertia=[75.153076467382206 23.577652078949701 94.231108050856861]  MomentsOfInertiaUnits=kg*mm^2  ProductsOfInertia=[0.01532312637695204 0.0017211125494294708 -5.8798668472039237]  ProductsOfInertiaUnits=kg*mm^2  GraphicType=FromGeometry  MarkerShape=Sphere  MarkerSize=10  GraphicVisPropType=SimpleVisualProperties  GraphicDiffuseColor=[1.0 1.0 0.0]  GraphicOpacity=1  GraphicSpecularColor=[0.5 0.5 0.5 1.0]  GraphicAmbientColor=[0.15 0.15 0.15 1.0]  GraphicEmissiveColor=[0.0 0.0 0.0 1.0]  GraphicShininess=75  DoExposeReferenceFrame=on  SerializedFrames=<Frames/>
  F : PMIOPort  Side=Left
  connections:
  Solid/RConn1 -- ReferenceFrame/RConn1 -- F/RConn1

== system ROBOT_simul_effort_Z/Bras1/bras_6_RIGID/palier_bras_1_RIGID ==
  ReferenceFrame : sm_lib/Frames and Transforms/Reference Frame
  Solid : sm_lib/Body Elements/File Solid  ExtGeomFileName=/MATLAB Drive/Fichiers_Matlab_sujetA/Fichiers Matlab/STL/palier bras_Defaut_sldprt.STL  UnitType=Custom  ExtGeomFileUnits=mm  StepReaderType=HEX  ExportConvexHullGeometry=off  InertiaType=Custom  BasedOnType=Density  Density=1000  DensityUnits=kg/(m^3)  Mass=0.00017920168094851793  MassUnits=kg  CenterOfMass=[-178.32667601154176 39.825618202078154 -20.980989744703667]  CenterOfMassUnits=mm  MomentsOfInertia=[0.0018602253674838991 0.0012789874237151958 0.0012789874237151961]  MomentsOfInertiaUnits=kg*mm^2  ProductsOfInertia=[0 0 0]  ProductsOfInertiaUnits=kg*mm^2  GraphicType=FromGeometry  MarkerShape=Sphere  MarkerSize=10  GraphicVisPropType=SimpleVisualProperties  GraphicDiffuseColor=[1 1 1]  GraphicOpacity=1  GraphicSpecularColor=[0.5 0.5 0.5 1.0]  GraphicAmbientColor=[0.15 0.15 0.15 1.0]  GraphicEmissiveColor=[0.0 0.0 0.0 1.0]  GraphicShininess=75  DoExposeReferenceFrame=on  SerializedFrames=<Frames/>
  F : PMIOPort  Side=Left
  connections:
  Solid/RConn1 -- ReferenceFrame/RConn1 -- F/RConn1

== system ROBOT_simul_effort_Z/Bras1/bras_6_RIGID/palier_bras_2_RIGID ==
  ReferenceFrame : sm_lib/Frames and Transforms/Reference Frame
  Solid : sm_lib/Body Elements/File Solid  ExtGeomFileName=/MATLAB Drive/Fichiers_Matlab_sujetA/Fichiers Matlab/STL/palier bras_Defaut_sldprt.STL  UnitType=Custom  ExtGeomFileUnits=mm  StepReaderType=HEX  ExportConvexHullGeometry=off  InertiaType=Custom  BasedOnType=Density  Density=1000  DensityUnits=kg/(m^3)  Mass=0.00017920168094851793  MassUnits=kg  CenterOfMass=[-178.32667601154176 39.825618202078154 -20.980989744703667]  CenterOfMassUnits=mm  MomentsOfInertia=[0.0018602253674838991 0.0012789874237151958 0.0012789874237151961]  MomentsOfInertiaUnits=kg*mm^2  ProductsOfInertia=[0 0 0]  ProductsOfInertiaUnits=kg*mm^2  GraphicType=FromGeometry  MarkerShape=Sphere  MarkerSize=10  GraphicVisPropType=SimpleVisualProperties  GraphicDiffuseColor=[1 1 1]  GraphicOpacity=1  GraphicSpecularColor=[0.5 0.5 0.5 1.0]  GraphicAmbientColor=[0.15 0.15 0.15 1.0]  GraphicEmissiveColor=[0.0 0.0 0.0 1.0]  GraphicShininess=75  DoExposeReferenceFrame=on  SerializedFrames=<Frames/>
  F : PMIOPort  Side=Left
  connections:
  Solid/RConn1 -- ReferenceFrame/RConn1 -- F/RConn1

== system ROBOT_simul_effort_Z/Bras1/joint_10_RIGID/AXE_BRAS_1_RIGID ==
  ReferenceFrame : sm_lib/Frames and Transforms/Reference Frame
  Solid : sm_lib/Body Elements/File Solid  ExtGeomFileName=/MATLAB Drive/Fichiers_Matlab_sujetA/Fichiers Matlab/STL/AXE BRAS_Defaut_sldprt.STL  UnitType=Custom  ExtGeomFileUnits=mm  StepReaderType=HEX  ExportConvexHullGeometry=off  InertiaType=Custom  BasedOnType=Density  Density=1000  DensityUnits=kg/(m^3)  Mass=0.0015327306958088996  MassUnits=kg  CenterOfMass=[0 0 0]  CenterOfMassUnits=mm  MomentsOfInertia=[0.11359646260705632 0.11359646260705632 0.0017137152305883286]  MomentsOfInertiaUnits=kg*mm^2  ProductsOfInertia=[0 0 0]  ProductsOfInertiaUnits=kg*mm^2  GraphicType=FromGeometry  MarkerShape=Sphere  MarkerSize=10  GraphicVisPropType=SimpleVisualProperties  GraphicDiffuseColor=[0.6470588235294118 0.61960784313725492 0.58823529411764708]  GraphicOpacity=1  GraphicSpecularColor=[0.5 0.5 0.5 1.0]  GraphicAmbientColor=[0.15 0.15 0.15 1.0]  GraphicEmissiveColor=[0.0 0.0 0.0 1.0]  GraphicShininess=75  DoExposeReferenceFrame=on  SerializedFrames=<Frames/>
  F : PMIOPort  Side=Left
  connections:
  Solid/RConn1 -- ReferenceFrame/RConn1 -- F/RConn1

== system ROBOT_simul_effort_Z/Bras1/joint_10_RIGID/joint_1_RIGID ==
  ReferenceFrame : sm_lib/Frames and Transforms/Reference Frame
  Solid : sm_lib/Body Elements/File Solid  ExtGeomFileName=/MATLAB Drive/Fichiers_Matlab_sujetA/Fichiers Matlab/STL/joint_Defaut_sldprt.STL  UnitType=Custom  ExtGeomFileUnits=mm  StepReaderType=HEX  ExportConvexHullGeometry=off  InertiaType=Custom  BasedOnType=Density  Density=1000  DensityUnits=kg/(m^3)  Mass=0.0062454336323428689  MassUnits=kg  CenterOfMass=[-4.7519597301086606e-06 14.873568128586268 0.2827021501004604]  CenterOfMassUnits=mm  MomentsOfInertia=[0.43544209184236687 0.81590742360241675 0.91424830357082487]  MomentsOfInertiaUnits=kg*mm^2  ProductsOfInertia=[0.0068320776316595647 -4.173068650825101e-06 -7.5142319098046527e-07]  ProductsOfInertiaUnits=kg*mm^2  GraphicType=FromGeometry  MarkerShape=Sphere  MarkerSize=10  GraphicVisPropType=SimpleVisualProperties  GraphicDiffuseColor=[1 1 1]  GraphicOpacity=1  GraphicSpecularColor=[0.5 0.5 0.5 1.0]  GraphicAmbientColor=[0.15 0.15 0.15 1.0]  GraphicEmissiveColor=[0.0 0.0 0.0 1.0]  GraphicShininess=75  DoExposeReferenceFrame=on  SerializedFrames=<Frames/>
  F : PMIOPort  Side=Left
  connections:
  Solid/RConn1 -- ReferenceFrame/RConn1 -- F/RConn1

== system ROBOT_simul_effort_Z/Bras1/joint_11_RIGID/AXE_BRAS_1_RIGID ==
  ReferenceFrame : sm_lib/Frames and Transforms/Reference Frame
  Solid : sm_lib/Body Elements/File Solid  ExtGeomFileName=/MATLAB Drive/Fichiers_Matlab_sujetA/Fichiers Matlab/STL/AXE BRAS_Defaut_sldprt.STL  UnitType=Custom  ExtGeomFileUnits=mm  StepReaderType=HEX  ExportConvexHullGeometry=off  InertiaType=Custom  BasedOnType=Density  Density=1000  DensityUnits=kg/(m^3)  Mass=0.0015327306958088996  MassUnits=kg  CenterOfMass=[0 0 0]  CenterOfMassUnits=mm  MomentsOfInertia=[0.11359646260705632 0.11359646260705632 0.0017137152305883286]  MomentsOfInertiaUnits=kg*mm^2  ProductsOfInertia=[0 0 0]  ProductsOfInertiaUnits=kg*mm^2  GraphicType=FromGeometry  MarkerShape=Sphere  MarkerSize=10  GraphicVisPropType=SimpleVisualProperties  GraphicDiffuseColor=[0.6470588235294118 0.61960784313725492 0.58823529411764708]  GraphicOpacity=1  GraphicSpecularColor=[0.5 0.5 0.5 1.0]  GraphicAmbientColor=[0.15 0.15 0.15 1.0]  GraphicEmissiveColor=[0.0 0.0 0.0 1.0]  GraphicShininess=75  DoExposeReferenceFrame=on  SerializedFrames=<Frames/>
  F : PMIOPort  Side=Left
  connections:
  Solid/RConn1 -- ReferenceFrame/RConn1 -- F/RConn1

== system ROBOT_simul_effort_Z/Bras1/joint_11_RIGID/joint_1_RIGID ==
  ReferenceFrame : sm_lib/Frames and Transforms/Reference Frame
  Solid : sm_lib/Body Elements/File Solid  ExtGeomFileName=/MATLAB Drive/Fichiers_Matlab_sujetA/Fichiers Matlab/STL/joint_Defaut_sldprt.STL  UnitType=Custom  ExtGeomFileUnits=mm  StepReaderType=HEX  ExportConvexHullGeometry=off  InertiaType=Custom  BasedOnType=Density  Density=1000  DensityUnits=kg/(m^3)  Mass=0.0062454336323428689  MassUnits=kg  CenterOfMass=[-4.7519597301086606e-06 14.873568128586268 0.2827021501004604]  CenterOfMassUnits=mm  MomentsOfInertia=[0.43544209184236687 0.81590742360241675 0.91424830357082487]  MomentsOfInertiaUnits=kg*mm^2  ProductsOfInertia=[0.0068320776316595647 -4.173068650825101e-06 -7.5142319098046527e-07]  ProductsOfInertiaUnits=kg*mm^2  GraphicType=FromGeometry  MarkerShape=Sphere  MarkerSize=10  GraphicVisPropType=SimpleVisualProperties  GraphicDiffuseColor=[1 1 1]  GraphicOpacity=1  GraphicSpecularColor=[0.5 0.5 0.5 1.0]  GraphicAmbientColor=[0.15 0.15 0.15 1.0]  GraphicEmissiveColor=[0.0 0.0 0.0 1.0]  GraphicShininess=75  DoExposeReferenceFrame=on  SerializedFrames=<Frames/>
  F : PMIOPort  Side=Left
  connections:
  Solid/RConn1 -- ReferenceFrame/RConn1 -- F/RConn1

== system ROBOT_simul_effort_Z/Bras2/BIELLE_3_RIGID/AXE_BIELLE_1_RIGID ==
  ReferenceFrame : sm_lib/Frames and Transforms/Reference Frame
  Solid : sm_lib/Body Elements/File Solid  ExtGeomFileName=/MATLAB Drive/Fichiers_Matlab_sujetA/Fichiers Matlab/STL/AXE BIELLE_Defaut_sldprt.STL  UnitType=Custom  ExtGeomFileUnits=mm  StepReaderType=HEX  ExportConvexHullGeometry=off  InertiaType=Custom  BasedOnType=Density  Density=1000  DensityUnits=kg/(m^3)  Mass=0.0008880235381781051  MassUnits=kg  CenterOfMass=[0 0 0]  CenterOfMassUnits=mm  MomentsOfInertia=[0.018768660222737772 0.018768660222737772 0.0009874025874388381]  MomentsOfInertiaUnits=kg*mm^2  ProductsOfInertia=[0 0 0]  ProductsOfInertiaUnits=kg*mm^2  GraphicType=FromGeometry  MarkerShape=Sphere  MarkerSize=10  GraphicVisPropType=SimpleVisualProperties  GraphicDiffuseColor=[1 0.94901960784313721 0.90980392156862744]  GraphicOpacity=1  GraphicSpecularColor=[0.5 0.5 0.5 1.0]  GraphicAmbientColor=[0.15 0.15 0.15 1.0]  GraphicEmissiveColor=[0.0 0.0 0.0 1.0]  GraphicShininess=75  DoExposeReferenceFrame=on  SerializedFrames=<Frames/>
  F : PMIOPort  Side=Left
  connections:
  Solid/RConn1 -- ReferenceFrame/RConn1 -- F/RConn1

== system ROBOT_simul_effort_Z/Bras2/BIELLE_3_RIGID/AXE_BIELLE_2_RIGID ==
  ReferenceFrame : sm_lib/Frames and Transforms/Reference Frame
  Solid : sm_lib/Body Elements/File Solid  ExtGeomFileName=/MATLAB Drive/Fichiers_Matlab_sujetA/Fichiers Matlab/STL/AXE BIELLE_Defaut_sldprt.STL  UnitType=Custom  ExtGeomFileUnits=mm  StepReaderType=HEX  ExportConvexHullGeometry=off  InertiaType=Custom  BasedOnType=Density  Density=1000  DensityUnits=kg/(m^3)  Mass=0.0008880235381781051  MassUnits=kg  CenterOfMass=[0 0 0]  CenterOfMassUnits=mm  MomentsOfInertia=[0.018768660222737772 0.018768660222737772 0.0009874025874388381]  MomentsOfInertiaUnits=kg*mm^2  ProductsOfInertia=[0 0 0]  ProductsOfInertiaUnits=kg*mm^2  GraphicType=FromGeometry  MarkerShape=Sphere  MarkerSize=10  GraphicVisPropType=SimpleVisualProperties  GraphicDiffuseColor=[1 0.94901960784313721 0.90980392156862744]  GraphicOpacity=1  GraphicSpecularColor=[0.5 0.5 0.5 1.0]  GraphicAmbientColor=[0.15 0.15 0.15 1.0]  GraphicEmissiveColor=[0.0 0.0 0.0 1.0]  GraphicShininess=75  DoExposeReferenceFrame=on  SerializedFrames=<Frames/>
  F : PMIOPort  Side=Left
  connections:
  Solid/RConn1 -- ReferenceFrame/RConn1 -- F/RConn1

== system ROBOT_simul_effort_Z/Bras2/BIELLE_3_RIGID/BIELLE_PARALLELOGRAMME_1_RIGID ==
  ReferenceFrame : sm_lib/Frames and Transforms/Reference Frame
  Solid : sm_lib/Body Elements/File Solid  ExtGeomFileName=/MATLAB Drive/Fichiers_Matlab_sujetA/Fichiers Matlab/STL/BIELLE PARALLELOGRAMME_Defaut_sldprt.STL  UnitType=Custom  ExtGeomFileUnits=mm  StepReaderType=HEX  ExportConvexHullGeometry=off  InertiaType=Custom  BasedOnType=Density  Density=1000  DensityUnits=kg/(m^3)  Mass=0.0079529027635324764  MassUnits=kg  CenterOfMass=[0 3.1653377955585489 0]  CenterOfMassUnits=mm  MomentsOfInertia=[7.7987017961340088 7.8475939194203406 0.14816857834406802]  MomentsOfInertiaUnits=kg*mm^2  ProductsOfInertia=[0 0 0]  ProductsOfInertiaUnits=kg*mm^2  GraphicType=FromGeometry  MarkerShape=Sphere  MarkerSize=10  GraphicVisPropType=SimpleVisualProperties  GraphicDiffuseColor=[0.6 1.0 1.0]  GraphicOpacity=1  GraphicSpecularColor=[0.5 0.5 0.5 1.0]  GraphicAmbientColor=[0.15 0.15 0.15 1.0]  GraphicEmissiveColor=[0.0 0.0 0.0 1.0]  GraphicShininess=75  DoExposeReferenceFrame=on  SerializedFrames=<Frames/>
  F : PMIOPort  Side=Left
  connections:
  Solid/RConn1 -- ReferenceFrame/RConn1 -- F/RConn1

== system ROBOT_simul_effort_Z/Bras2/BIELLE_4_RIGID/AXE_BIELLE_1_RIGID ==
  ReferenceFrame : sm_lib/Frames and Transforms/Reference Frame
  Solid : sm_lib/Body Elements/File Solid  ExtGeomFileName=/MATLAB Drive/Fichiers_Matlab_sujetA/Fichiers Matlab/STL/AXE BIELLE_Defaut_sldprt.STL  UnitType=Custom  ExtGeomFileUnits=mm  StepReaderType=HEX  ExportConvexHullGeometry=off  InertiaType=Custom  BasedOnType=Density  Density=1000  DensityUnits=kg/(m^3)  Mass=0.0008880235381781051  MassUnits=kg  CenterOfMass=[0 0 0]  CenterOfMassUnits=mm  MomentsOfInertia=[0.018768660222737772 0.018768660222737772 0.0009874025874388381]  MomentsOfInertiaUnits=kg*mm^2  ProductsOfInertia=[0 0 0]  ProductsOfInertiaUnits=kg*mm^2  GraphicType=FromGeometry  MarkerShape=Sphere  MarkerSize=10  GraphicVisPropType=SimpleVisualProperties  GraphicDiffuseColor=[1 0.94901960784313721 0.90980392156862744]  GraphicOpacity=1  GraphicSpecularColor=[0.5 0.5 0.5 1.0]  GraphicAmbientColor=[0.15 0.15 0.15 1.0]  GraphicEmissiveColor=[0.0 0.0 0.0 1.0]  GraphicShininess=75  DoExposeReferenceFrame=on  SerializedFrames=<Frames/>
  F : PMIOPort  Side=Left
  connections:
  Solid/RConn1 -- ReferenceFrame/RConn1 -- F/RConn1
